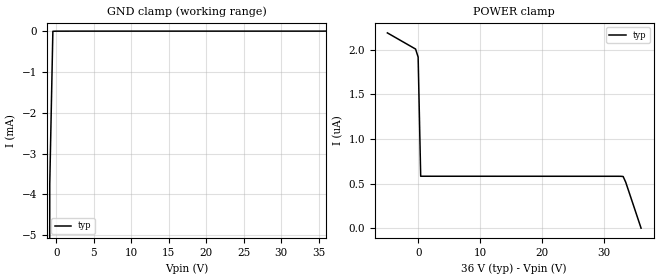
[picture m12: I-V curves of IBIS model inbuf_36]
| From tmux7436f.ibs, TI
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| inbuf_36
[Model]   inbuf_36
Model_type   Input
Vinl = 0.8
Vinh = 1.3
|   typ   min   max
C_comp   6.362683e-13   NA   NA
[Voltage Range]   36   NA   NA
[Temperature Range]   27   NA   NA
[Power Clamp Reference]   36   NA   NA
[GND Clamp Reference]   0   NA   NA
[GND Clamp]
|   Voltage   I(typ)   I(min)   I(max)
-5V       -1.962A    NA         NA
-1.273V   -119.9mA   NA         NA
-858.6mV  -3.749mA   NA         NA
-444.4mV  -3.246uA   NA         NA
36V       1.792uA    NA         NA
[POWER Clamp]
|   Voltage   I(typ)   I(min)   I(max)
-5V       2.188uA    NA         NA
-444.4mV  2.007uA    NA         NA
-30.3mV   1.917uA    NA         NA
383.8mV   581.7nA    NA         NA
33.1V     579nA      NA         NA
33.52V    515.7nA    NA         NA
36V       -196.9pA   NA         NA
